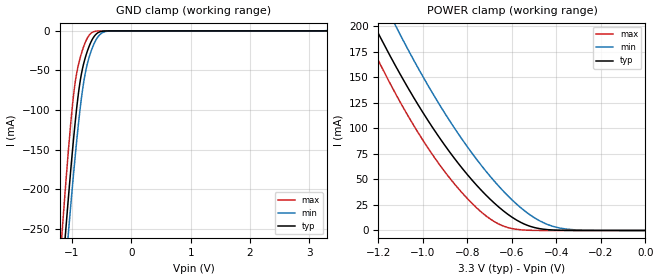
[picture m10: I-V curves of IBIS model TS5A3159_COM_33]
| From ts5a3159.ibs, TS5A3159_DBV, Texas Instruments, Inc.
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[Model]   TS5A3159_COM_33
Model_type  Terminator
| variable   typ   min   max
C_comp   47.94pF   38.11pF   54.99pF
| C_tri-state   47.94pF   38.11pF   54.99pF
[Temperature Range]   40   100   -40
| Ambient temperature   25   85   -40
[Voltage range]   3.3   3   3.6
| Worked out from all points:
|   GND clamp passes 1 mA (typ) near -0.52 V on its own axis
|   POWER clamp passes 1 mA (typ) near -0.45 V on its own axis
[GND Clamp]
| TS5A3159_COM_33
|   Voltage   I(typ)   I(min)   I(max)
-3.3V     -2.932A    -2.86A     -3.058A
-1.17V    -314mA     -356.6mA   -257.3mA
-1.12V    -265.6mA   -309.4mA   -207.1mA
-1.095V   -242.1mA   -286.4mA   -182.9mA
-1.055V   -205.5mA   -250.2mA   -145.8mA
-935mV    -107.1mA   -149.7mA   -59.35mA
-870mV    -67.19mA   -102.9mA   -36.23mA
-800mV    -40.32mA   -63.41mA   -19.01mA
-655mV    -10.3mA    -20.97mA   -1.712mA
-535mV    -1.288mA   -5.005mA   -49.9uA
-360mV    -12.77uA   -150.1uA   -49.23nA
3.3V      4.479nA    423.9uA    3.532nA
[POWER Clamp]
| TS5A3159_COM_33
|   Voltage   I(typ)   I(min)   I(max)
-3.3V     1.645A     1.724A     1.734A
-1.275V   225.2mA    269.3mA    199.9mA
-1.21V    196.6mA    238.8mA    170.3mA
-1.125V   161.6mA    201.1mA    134.5mA
-1.105V   153.8mA    192.6mA    126.5mA
-960mV    101.7mA    135.4mA    75mA
-800mV    54.51mA    81.68mA    31.11mA
-680mV    26.89mA    48.37mA    8.728mA
-545mV    6.306mA    19.52mA    425.4uA
-455mV    1.141mA    7.226mA    22.26uA
-385mV    209uA      2.361mA    1.548uA
0V        0A         0A         0A
